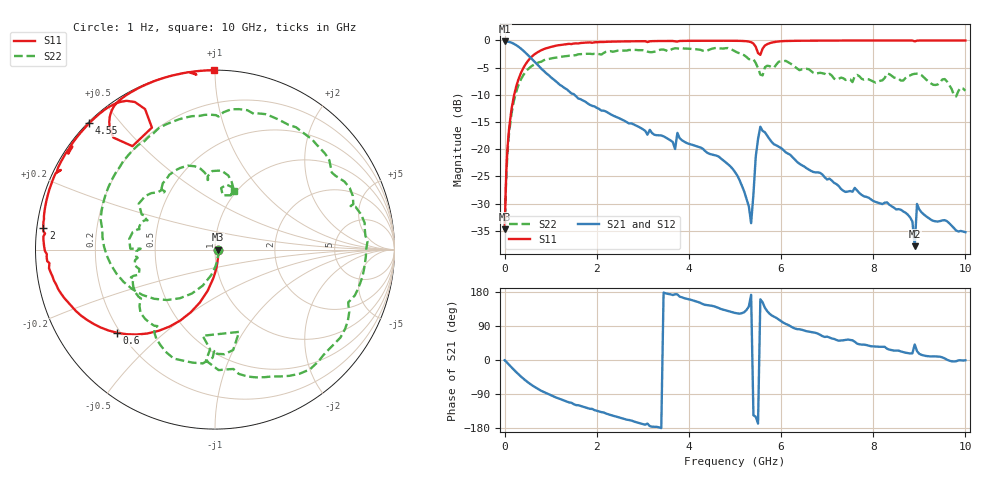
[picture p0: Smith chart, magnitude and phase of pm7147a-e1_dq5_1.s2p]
# GHz S DB R 50
! S-Parameters data
! Freq  dbS11  angS11  dbS21  angS21  dbS12  angS12  dbS22  angS22
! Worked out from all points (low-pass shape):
!   279 points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, 1 Hz to 10 GHz, reference 50 ohm
!   highest |S21| = -0.16 dB at 6.31 kHz (marker M1); lowest = -37.8 dB at 8.9 GHz (marker M2)
!   |S21| within 3 dB of the highest: start of sweep to 562 MHz
!   lowest |S11| = -34.7 dB at 6.31 kHz (marker M3), VSWR 1.04, Z = 51.9 - j0.000935 ohm
!   |S11| at or under -10 dB: start of sweep to 207.9 MHz
!   |S22| runs from -34.7 to -1.4 dB; largest |S21 - S12| = 4e-13
!   S11 on the Smith chart (normalised r, x): 1 Hz: 1.04, -0.00; 600 MHz: 0.19, -0.36; 2 GHz: 0.02, +0.06; 4.55 GHz: 0.00, +0.42; 10 GHz: 0.00, +0.99
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1e-09  -34.73 -0.0  -0.16 0.0  -0.16 0.0  -34.73 -0.0
6.3096e-06  -34.73 -0.0  -0.16 -0.0  -0.16 -0.0  -34.73 -0.0
0.05011872  -21.75 -81.7  -0.19 -6.5  -0.19 -6.5  -22.50 -83.5
0.15  -12.61 -100.2  -0.42 -19.4  -0.42 -19.4  -13.45 -108.9
0.6  -2.90 -139.7  -3.49 -67.0  -3.49 -67.0  -4.64 -171.7
1  -1.20 -160.4  -6.74 -92.9  -6.74 -92.9  -3.32 153.3
1.7  -0.43 179.1  -11.04 -123.3  -11.04 -123.3  -2.49 108.3
2  -0.31 172.8  -12.39 -134.0  -12.39 -134.0  -2.48 91.9
3.35  -0.11 150.6  -17.43 -177.7  -17.43 -177.7  -1.77 27.6
4.55  -0.06 134.8  -21.08 141.5  -21.08 141.5  -1.42 -31.2
5.05  -0.07 127.8  -24.83 123.1  -24.83 123.1  -2.22 -65.7
5.35  -0.32 120.7  -33.59 172.1  -33.59 172.1  -3.46 -83.0
5.45  -1.16 116.5  -21.40 -149.8  -21.40 -149.8  -4.14 -94.7
5.55  -2.65 128.6  -15.85 160.1  -15.85 160.1  -6.29 -98.1
5.6  -1.49 132.2  -16.63 152.0  -16.63 152.0  -6.42 -73.7
6  -0.15 123.9  -19.78 102.4  -19.78 102.4  -3.85 -101.3
6.7  -0.04 115.6  -24.17 72.6  -24.17 72.6  -5.96 -145.7
8.35  -0.01 101.5  -30.20 27.4  -30.20 27.4  -6.20 142.3
8.8  -0.01 98.0  -32.52 17.2  -32.52 17.2  -6.43 124.5
8.9  -0.17 96.1  -37.81 40.9  -37.81 40.9  -6.14 116.2
8.95  -0.04 97.9  -30.05 23.3  -30.05 23.3  -6.11 113.2
10  -0.00 90.3  -35.24 -0.7  -35.24 -0.7  -9.25 72.6
